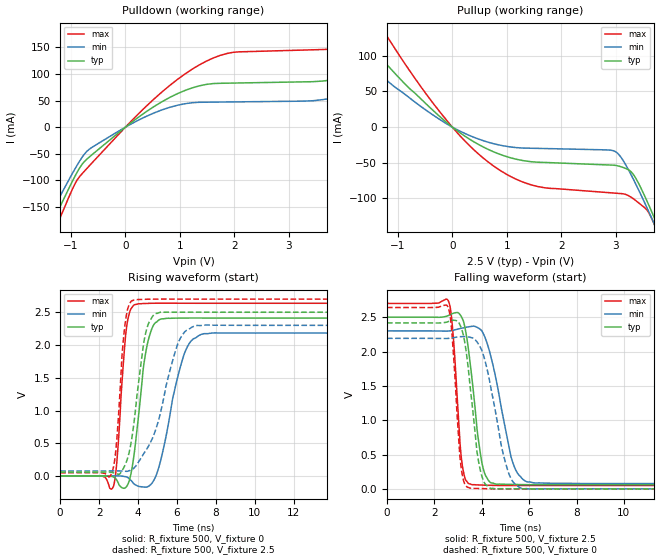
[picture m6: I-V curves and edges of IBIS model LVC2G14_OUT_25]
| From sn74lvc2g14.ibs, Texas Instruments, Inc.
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[Model]   LVC2G14_OUT_25
Model_type  Output
Vref =   0
Rref =   500
Cref =   30p
Vmeas =   1.25
| variable   typ   min   max
C_comp   9.70pF   6.16pF   13.61pF
| C_pullup   9.66pF   6.16pF   11.44pF
| C_pulldown   9.73pF   6.26pF   13.61pF
[Temperature Range]   40   100   -40
| Ambient temperature   25   85   -40
[Voltage range]   2.5   2.3   2.7
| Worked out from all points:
|   slope of the pulldown table from 0 to 0.375 V, typ, clamps not added: 13.1 ohm
|   slope of the pullup table from 0 to 0.375 V, typ, clamps not added: 19 ohm
|   rising waveform, R_fixture 500, V_fixture 0: 20-80 % time 561ps typ, 934ps min, 360ps max; typ from 0 V to 2.41 V
|   falling waveform, R_fixture 500, V_fixture 2.5: 20-80 % time 483ps typ, 767ps min, 295ps max; typ from 2.5 V to 0.06 V
|   rising waveform, R_fixture 500, V_fixture 2.5: 20-80 % time 617ps typ, 1.22ns min, 360ps max; typ from 0.06 V to 2.5 V
|   falling waveform, R_fixture 500, V_fixture 0: 20-80 % time 458ps typ, 739ps min, 291ps max; typ from 2.42 V to 0 V
[Pulldown]
| LVC2G14_OUT_25
|   Voltage   I(typ)   I(min)   I(max)
-5.5V     -1.065A    -962.2mA   -1.199A
-1.53V    -221.1mA   -193.8mA   -251.2mA
-1.17V    -142.7mA   -123.7mA   -162.8mA
-670mV    -56.67mA   -41.91mA   -73.36mA
520mV     38.43mA    26.46mA    52.49mA
1.485V    80.34mA    46.87mA    124mA
3.84V     90.07mA    55.63mA    147.9mA
5.34V     157.5mA    105.9mA    231.4mA
5.91V     188.7mA    52.63mA    282.8mA
6.525V    93.57mA    53.14mA    298.9mA
7.56V     94.12mA    54.12mA    160.7mA
11V       99.65mA    57.57mA    168.9mA
[Pullup]
| LVC2G14_OUT_25
|   Voltage   I(typ)   I(min)   I(max)
-5.5V     533.4mA    418.6mA    746.4mA
-2.34V    192.7mA    147.4mA    275.6mA
-1.735V   134.9mA    102mA      194.6mA
-1.32V    97.81mA    73.23mA    142.1mA
-135mV    8.418mA    6.055mA    12.49mA
750mV     -34.38mA   -23.05mA   -54.11mA
1.57V     -49.22mA   -29.81mA   -83.34mA
2.995V    -53.63mA   -34.3mA    -92.61mA
3.315V    -65.3mA    -71.46mA   -99.87mA
3.565V    -101.9mA   -111.4mA   -115.4mA
3.75V     -134.3mA   -142.6mA   -143.5mA
11V       -1.614A    -1.516A    -1.761A
[Ramp]
| LVC2G14_OUT_25
| variable   typ   min   max
dV/dt_r   1.56/6.52E-10   1.41/1.04E-09   1.70/3.91E-10
dV/dt_f   1.50/5.31E-10   1.38/8.05E-10   1.63/3.12E-10
R_load = 500
[Rising Waveform]
| LVC2G14_OUT_25
R_fixture =   500
C_fixture =   0
L_fixture =   0
V_fixture =   0
V_fixture_min = 0
V_fixture_max = 0
|   Time   V(typ)   V(min)   V(max)
0s        123.6pV    5.747nV    2.756nV
2.725ns   -13.51mV   1.352mV    -166mV
2.92ns    -67.9mV    1.562mV    245.7mV
3.38ns    -171.7mV   -11.87mV   2.195V
3.835ns   415.8mV    -129.4mV   2.617V
4.32ns    1.746V     -168.7mV   2.634V
4.775ns   2.292V     -83.17mV   2.637V
6.365ns   2.412V     1.858V     2.637V
7.255ns   2.412V     2.163V     2.637V
24.99ns   2.411V     2.183V     2.637V
[Falling Waveform]
| LVC2G14_OUT_25
R_fixture =   500
C_fixture =   0
L_fixture =   0
V_fixture =   2.5
V_fixture_min = 2.3
V_fixture_max = 2.7
|   Time   V(typ)   V(min)   V(max)
0s        2.5V       2.3V       2.7V
2.59ns    2.524V     2.298V     2.736V
2.77ns    2.552V     2.307V     2.326V
3.145ns   2.502V     2.338V     432.3mV
3.465ns   1.957V     2.36V      73.46mV
3.855ns   722.4mV    2.342V     57.7mV
4.15ns    201.4mV    2.192V     54.02mV
5.245ns   65.73mV    454.9mV    48.94mV
5.9ns     61.66mV    104.7mV    49mV
24.99ns   60.11mV    77.11mV    49.35mV
[Rising Waveform]
| LVC2G14_OUT_25
R_fixture =   500
C_fixture =   0
L_fixture =   0
V_fixture =   2.5
V_fixture_min = 2.3
V_fixture_max = 2.7
|   Time   V(typ)   V(min)   V(max)
0s        60.06mV    77.04mV    49.31mV
2.64ns    55.97mV    77.9mV     36.22mV
2.885ns   35.12mV    78.29mV    469.9mV
3.31ns    152.5mV    73.66mV    2.261V
3.695ns   603.6mV    101.6mV    2.678V
4.29ns    2.03V      340.5mV    2.697V
4.57ns    2.348V     473.4mV    2.699V
6.025ns   2.5V       2.005V     2.7V
6.89ns    2.501V     2.289V     2.7V
24.99ns   2.5V       2.3V       2.7V
[Falling Waveform]
| LVC2G14_OUT_25
R_fixture =   500
C_fixture =   0
L_fixture =   0
V_fixture =   0
V_fixture_min = 0
V_fixture_max = 0
|   Time   V(typ)   V(min)   V(max)
0s        2.416V     2.191V     2.64V
2.575ns   2.434V     2.19V      2.646V
2.74ns    2.451V     2.197V     2.265V
3.12ns    2.354V     2.216V     333.7mV
3.495ns   1.536V     2.208V     12.52mV
3.795ns   549.3mV    2.141V     6.828mV
4.095ns   99.98mV    1.917V     3.584mV
5.035ns   3.081mV    339.6mV    -297.5uV
5.695ns   1.068mV    6.234mV    -298uV
24.99ns   42.17uV    58.79uV    35.63uV
